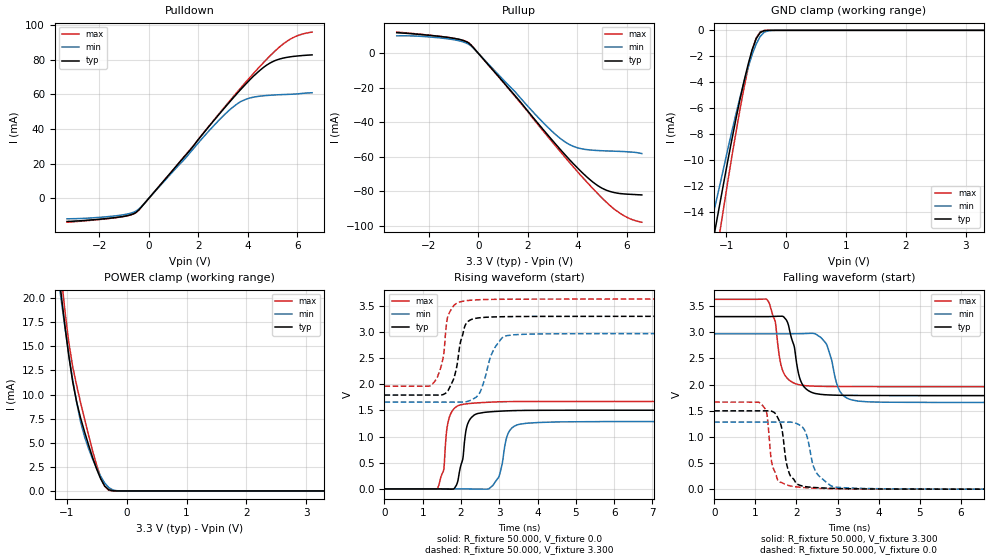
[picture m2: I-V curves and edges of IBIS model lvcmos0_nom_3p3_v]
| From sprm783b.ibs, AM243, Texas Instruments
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|   nom_3p3_v
[Model]   lvcmos0_nom_3p3_v
Model_type I/O
Polarity   Non-Inverting
Enable   Active-High
Vinl = 0
Vinh = 0.8
Vmeas = 1.65
Vref = 3.3
Cref = 2pF
Rref = 100000
|   typ   min   max
C_comp   3.777pF   3.679pF   3.786pF
[Voltage Range]   3.3   2.97   3.63
[Temperature Range]   27   150   -40
[Pullup Reference]   3.3   2.97   3.63
[Pulldown Reference]   0   0   0
[Power Clamp Reference]   3.3   2.97   3.63
[GND Clamp Reference]   0   0   0
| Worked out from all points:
|   slope of the pulldown table from 0 to 0.495 V, typ, clamps not added: 59.8 ohm
|   slope of the pullup table from 0 to 0.495 V, typ, clamps not added: 60.7 ohm
|   GND clamp passes 1 mA (typ) near -0.53 V on its own axis
|   POWER clamp passes 1 mA (typ) near -0.41 V on its own axis
|   rising waveform, R_fixture 50.000, V_fixture 0.0: 20-80 % time 204ps typ, 212ps min, 146ps max; typ from 0 V to 1.5 V
|   rising waveform, R_fixture 50.000, V_fixture 3.300: 20-80 % time 256ps typ, 350ps min, 194ps max; typ from 1.79 V to 3.3 V
|   falling waveform, R_fixture 50.000, V_fixture 3.300: 20-80 % time 250ps typ, 265ps min, 213ps max; typ from 3.3 V to 1.79 V
|   falling waveform, R_fixture 50.000, V_fixture 0.0: 20-80 % time 195ps typ, 293ps min, 178ps max; typ from 1.5 V to 0 V
[Pulldown]
|Voltage   I(typ)   I(min)   I(max)
-3.3V     -13.29mA   -11.75mA   -13.7mA
-1.4V     -11.12mA   -10.13mA   -11.23mA
-800mV    -9.721mA   -8.785mA   -9.805mA
-500mV    -7.931mA   -7.165mA   -8.018mA
1.6V      26.66mA    25.2mA     27mA
2.7V      46.1mA     43.08mA    46.41mA
3.6V      61.04mA    54.81mA    61.79mA
4V        67.16mA    57.58mA    68.4mA
4.4V      72.74mA    58.84mA    74.78mA
5V        78.87mA    59.63mA    83.67mA
5.8V      81.87mA    60.16mA    92.56mA
6.6V      82.83mA    60.99mA    95.99mA
[Pullup]
|Voltage   I(typ)   I(min)   I(max)
-3.3V     12mA       10.2mA     12.38mA
-1.4V     9.607mA    8.77mA     9.636mA
-800mV    8.234mA    7.423mA    8.249mA
-400mV    6.133mA    5.372mA    6.247mA
1V        -16.5mA    -15.2mA    -16.69mA
2.7V      -45.57mA   -41.35mA   -46.43mA
3.2V      -53.91mA   -48.06mA   -55.09mA
3.6V      -60.34mA   -52.22mA   -61.89mA
4.2V      -69.22mA   -55.4mA    -71.8mA
5V        -78.21mA   -56.44mA   -83.93mA
5.8V      -81.38mA   -56.87mA   -93.42mA
6.6V      -82.06mA   -58.07mA   -97.88mA
[GND_clamp]
|Voltage   I(typ)   I(min)   I(max)
-3.3V     -91.93mA   -62.08mA   -135.9mA
-1.3V     -18.16mA   -15.85mA   -21.32mA
-1.233V   -16.57mA   -14.51mA   -19.39mA
-1.167V   -14.92mA   -13.18mA   -17.39mA
-1.1V     -13.23mA   -11.81mA   -15.39mA
-1.033V   -11.55mA   -10.42mA   -13.42mA
-833mV    -6.742mA   -6.383mA   -7.774mA
-633mV    -2.616mA   -2.841mA   -2.875mA
-500mV    -654.1uA   -1.067mA   -592.9uA
-433mV    -179.7uA   -478.2uA   -124uA
-233mV    -333.7nA   -8.022uA   -209.7nA
3.3V      0A         0A         0A
[POWER_clamp]
|Voltage   I(typ)   I(min)   I(max)
-3.3V     163.7mA    143.3mA    185.7mA
-1.1V     20.75mA    20.14mA    22.78mA
-1.033V   17.24mA    17.07mA    18.82mA
-967mV    14.04mA    14.16mA    15.45mA
-900mV    11.29mA    11.5mA     12.86mA
-767mV    7.523mA    7.112mA    9.104mA
-633mV    4.713mA    4.344mA    5.707mA
-500mV    2.255mA    2.334mA    2.657mA
-367mV    510.2uA    822.4uA    470.8uA
-300mV    125.7uA    354.2uA    72.09uA
-100mV    199nA      4.751uA    105.3nA
3.3V      0A         0A         0A
[Ramp]
| variable   typ   min   max
dV/dt_r   0.903/0.203n   0.772/0.212n   1.003/0.146n
dV/dt_f   0.907/0.249n   0.787/0.264n   1.002/0.210n
R_load = 50.000
[Rising Waveform]
R_fixture= 50.000
V_fixture= 0.0
|time   V(typ)   V(min)   V(max)
0s        1.895uV    19.8uV     2.572uV
1.38ns    -155.4uV   24.41uV    4.525mV
1.549ns   -1.989mV   -115.2uV   369.3mV
1.68ns    -4.024mV   -24.52uV   1.332V
2.006ns   475.5mV    -280.6uV   1.61V
2.274ns   1.367V     -1.817mV   1.636V
2.831ns   1.478V     65.01mV    1.661V
3.222ns   1.493V     1.046V     1.669V
3.522ns   1.499V     1.235V     1.67V
10ns      1.504V     1.287V     1.672V
[Rising Waveform]
R_fixture= 50.000
V_fixture= 3.300
V_fixture_min= 2.970
V_fixture_max= 3.630
|time   V(typ)   V(min)   V(max)
0s        1.794V     1.659V     1.964V
1.254ns   1.794V     1.659V     2.003V
1.522ns   1.802V     1.659V     2.467V
1.624ns   1.847V     1.659V     3.178V
1.695ns   1.928V     1.659V     3.369V
2.034ns   2.92V      1.66V      3.586V
2.477ns   3.271V     1.824V     3.617V
2.857ns   3.288V     2.669V     3.624V
3.207ns   3.294V     2.932V     3.627V
10ns      3.3V       2.97V      3.63V
[Falling Waveform]
R_fixture= 50.000
V_fixture= 3.300
V_fixture_min= 2.970
V_fixture_max= 3.630
|time   V(typ)   V(min)   V(max)
0s        3.3V       2.97V      3.63V
1.284ns   3.3V       2.97V      3.627V
1.481ns   3.303V     2.97V      3.214V
1.617ns   3.307V     2.97V      2.4V
1.766ns   3.22V      2.97V      2.13V
2.074ns   2.14V      2.973V     1.995V
2.703ns   1.806V     2.804V     1.965V
3.041ns   1.796V     1.896V     1.962V
3.338ns   1.793V     1.708V     1.961V
10ns      1.789V     1.658V     1.96V
[Falling Waveform]
R_fixture= 50.000
V_fixture= 0.0
V_fixture_min= 0.0
V_fixture_max= 0.0
|time   V(typ)   V(min)   V(max)
0s        1.498V     1.283V     1.665V
1.144ns   1.498V     1.283V     1.631V
1.278ns   1.498V     1.283V     1.456V
1.432ns   1.479V     1.283V     410.2mV
1.63ns    1.209V     1.283V     127.7mV
1.858ns   247.9mV    1.282V     61.71mV
2.181ns   53.72mV    1.153V     30.18mV
2.467ns   30.54mV    339.9mV    17.76mV
2.89ns    15.12mV    48.25mV    9.097mV
10ns      66.8uV     145.2uV    36.97uV
